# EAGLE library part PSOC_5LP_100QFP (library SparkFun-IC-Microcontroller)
Cypress PSOC 5LP, 100-pin package We use the CY8C5868AXI-LP035, which has the "full" feature set: - 256k flash - 64k SRAM - 2k EEPROM - CAN - Full-speed USB - 67MHz operation Datasheet SparkFun Products FreeSoC2 Development Board - PSoC5LP (DEV-13229) -- Involved with change to new unposted revision
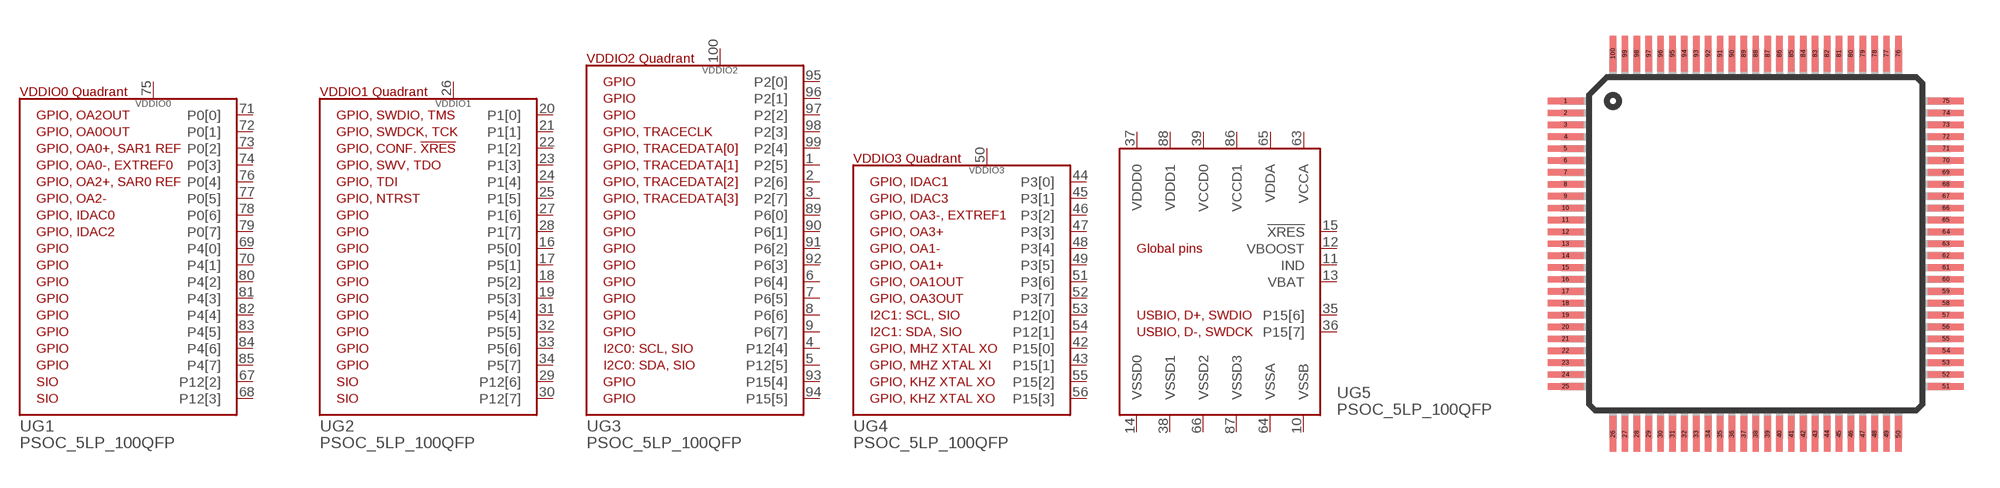
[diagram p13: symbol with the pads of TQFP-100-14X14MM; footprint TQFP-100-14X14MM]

Designator prefix U; gates G1=CY8C58LP_100QFP_VDDIO0 G2=CY8C58LP_100QFP_VDDIO1 G3=CY8C58LP_100QFP_VDDIO2 G4=CY8C58LP_100QFP_VDDIO3 G5=CY8C58LP_100QFP_VGLOBAL

## PSOC_5LP_100QFP (PROD_ID: IC-12190; VALUE: CY8C5868AXI-LP035)  [TQFP-100-14X14MM]
1  G3:P2[5]
2  G3:P2[6]
3  G3:P2[7]
4  G3:P12[4]
5  G3:P12[5]
6  G3:P6[4]
7  G3:P6[5]
8  G3:P6[6]
9  G3:P6[7]
10  G5:VSSB
11  G5:IND
12  G5:VBOOST
13  G5:VBAT
14  G5:VSSD0
15  G5:!XRES
16  G2:P5[0]
17  G2:P5[1]
18  G2:P5[2]
19  G2:P5[3]
20  G2:P1[0]
21  G2:P1[1]
22  G2:P1[2]
23  G2:P1[3]
24  G2:P1[4]
25  G2:P1[5]
26  G2:VDDIO1
27  G2:P1[6]
28  G2:P1[7]
29  G2:P12[6]
30  G2:P12[7]
31  G2:P5[4]
32  G2:P5[5]
33  G2:P5[6]
34  G2:P5[7]
35  G5:P15[6]
36  G5:P15[7]
37  G5:VDDD0
38  G5:VSSD1
39  G5:VCCD0
42  G4:P15[0]
43  G4:P15[1]
44  G4:P3[0]
45  G4:P3[1]
46  G4:P3[2]
47  G4:P3[3]
48  G4:P3[4]
49  G4:P3[5]
50  G4:VDDIO3
51  G4:P3[6]
52  G4:P3[7]
53  G4:P12[0]
54  G4:P12[1]
55  G4:P15[2]
56  G4:P15[3]
63  G5:VCCA
64  G5:VSSA
65  G5:VDDA
66  G5:VSSD2
67  G1:P12[2]
68  G1:P12[3]
69  G1:P4[0]
70  G1:P4[1]
71  G1:P0[0]
72  G1:P0[1]
73  G1:P0[2]
74  G1:P0[3]
75  G1:VDDIO0
76  G1:P0[4]
77  G1:P0[5]
78  G1:P0[6]
79  G1:P0[7]
80  G1:P4[2]
81  G1:P4[3]
82  G1:P4[4]
83  G1:P4[5]
84  G1:P4[6]
85  G1:P4[7]
86  G5:VCCD1
87  G5:VSSD3
88  G5:VDDD1
89  G3:P6[0]
90  G3:P6[1]
91  G3:P6[2]
92  G3:P6[3]
93  G3:P15[4]
94  G3:P15[5]
95  G3:P2[0]
96  G3:P2[1]
97  G3:P2[2]
98  G3:P2[3]
99  G3:P2[4]
100  G3:VDDIO2

## Footprint TQFP-100-14X14MM (pad centres in mm)
smd 1.5 x 0.27: 1 -8,6; 2 -8,5.5; 3 -8,5; 4 -8,4.5; 5 -8,4; 6 -8,3.5; 7 -8,3; 8 -8,2.5; 9 -8,2; 10 -8,1.5; 11 -8,1; 12 -8,0.5; 13 -8,0; 14 -8,-0.5; 15 -8,-1; 16 -8,-1.5; 17 -8,-2; 18 -8,-2.5; 19 -8,-3; 20 -8,-3.5; 21 -8,-4; 22 -8,-4.5; 23 -8,-5; 24 -8,-5.5; 25 -8,-6; 51 8,-6; 52 8,-5.5; 53 8,-5; 54 8,-4.5; 55 8,-4; 56 8,-3.5; 57 8,-3; 58 8,-2.5; 59 8,-2; 60 8,-1.5; 61 8,-1; 62 8,-0.5; 63 8,0; 64 8,0.5; 65 8,1; 66 8,1.5; 67 8,2; 68 8,2.5; 69 8,3; 70 8,3.5; 71 8,4; 72 8,4.5; 73 8,5; 74 8,5.5; 75 8,6
smd 0.27 x 1.5: 26 -6,-8; 27 -5.5,-8; 28 -5,-8; 29 -4.5,-8; 30 -4,-8; 31 -3.5,-8; 32 -3,-8; 33 -2.5,-8; 34 -2,-8; 35 -1.5,-8; 36 -1,-8; 37 -0.5,-8; 38 0,-8; 39 0.5,-8; 40 1,-8; 41 1.5,-8; 42 2,-8; 43 2.5,-8; 44 3,-8; 45 3.5,-8; 46 4,-8; 47 4.5,-8; 48 5,-8; 49 5.5,-8; 50 6,-8; 76 6,8; 77 5.5,8; 78 5,8; 79 4.5,8; 80 4,8; 81 3.5,8; 82 3,8; 83 2.5,8; 84 2,8; 85 1.5,8; 86 1,8; 87 0.5,8; 88 0,8; 89 -0.5,8; 90 -1,8; 91 -1.5,8; 92 -2,8; 93 -2.5,8; 94 -3,8; 95 -3.5,8; 96 -4,8; 97 -4.5,8; 98 -5,8; 99 -5.5,8; 100 -6,8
